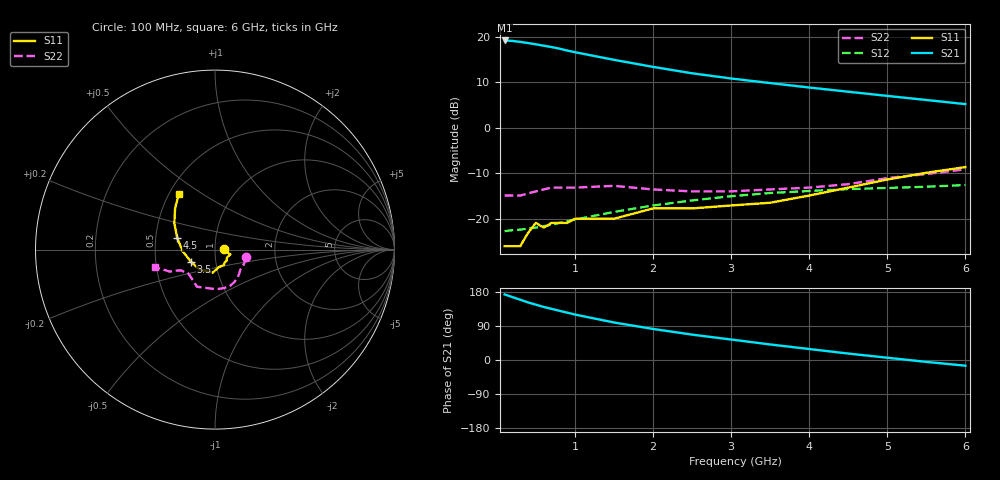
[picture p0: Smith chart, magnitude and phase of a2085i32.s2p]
!  MSA-2085 S AND NOISE PARAMETERS
!  Id = 32 mA  LAST UPDATED 06-27-94
# ghz s ma r 50
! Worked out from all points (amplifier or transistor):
!   20 points, 100 MHz to 6 GHz, reference 50 ohm
!   highest |S21| = 19.2 dB at 100 MHz (marker M1)
!   |S21| within 3 dB of that: start of sweep to 1.125 GHz
!   unconditionally stable (mu >= 1): start of sweep to end of sweep
!   at 400 MHz: K = 1.06, MAG = 18.9 dB, |S12| = -22.2 dB
!   at 1.5 GHz: K = 1.02, MAG = 15.9 dB, |S12| = -18.5 dB
!   at 6 GHz: K = 1.00, MAG = 8.8 dB, |S12| = -12.6 dB
!   S11 on the Smith chart (normalised r, x): 100 MHz: 1.10, +0.01; 3.5 GHz: 0.76, -0.11; 4.5 GHz: 0.65, +0.09; 6 GHz: 0.56, +0.40
0.1  0.05 4.0  9.11 173.0  0.073 4.0  0.18 -14.0
0.2  0.05 -6.0  9 166.0  0.075 8.0  0.18 -27.0
0.3  0.05 -14.0  8.79 159.0  0.076 11.0  0.18 -38.0
0.4  0.07 -13.0  8.53 152.0  0.078 14.0  0.19 -45.0
0.5  0.09 -17.0  8.26 146.0  0.08 17.0  0.2 -51.0
0.6  0.08 -33.0  7.98 140.0  0.083 19.0  0.21 -59.0
0.7  0.09 -44.0  7.71 135.0  0.086 22.0  0.22 -68.0
0.8  0.09 -47.0  7.41 130.0  0.09 24.0  0.22 -77.0
0.9  0.09 -54.0  7.06 125.0  0.094 26.0  0.22 -85.0
1  0.1 -60.0  6.77 120.0  0.098 27.0  0.22 -90.0
1.5  0.1 -78.0  5.58 99.0  0.119 31.0  0.23 -116.0
2  0.13 -96.0  4.67 82.0  0.14 31.0  0.21 -126.0
2.5  0.13 -113.0  3.97 67.0  0.159 30.0  0.2 -137.0
3  0.14 -129.0  3.48 54.0  0.177 27.0  0.2 -140.0
3.5  0.15 -153.0  3.1 41.0  0.192 24.0  0.21 -143.0
4  0.18 -177.0  2.77 29.0  0.202 22.0  0.22 -148.0
4.5  0.22 163.0  2.49 17.0  0.212 19.0  0.24 -151.0
5  0.27 147.0  2.24 6.0  0.218 17.0  0.28 -154.0
5.5  0.32 134.0  2.02 -5.0  0.225 15.0  0.31 -159.0
6  0.37 123.0  1.82 -15.0  0.235 14.0  0.35 -164.0
